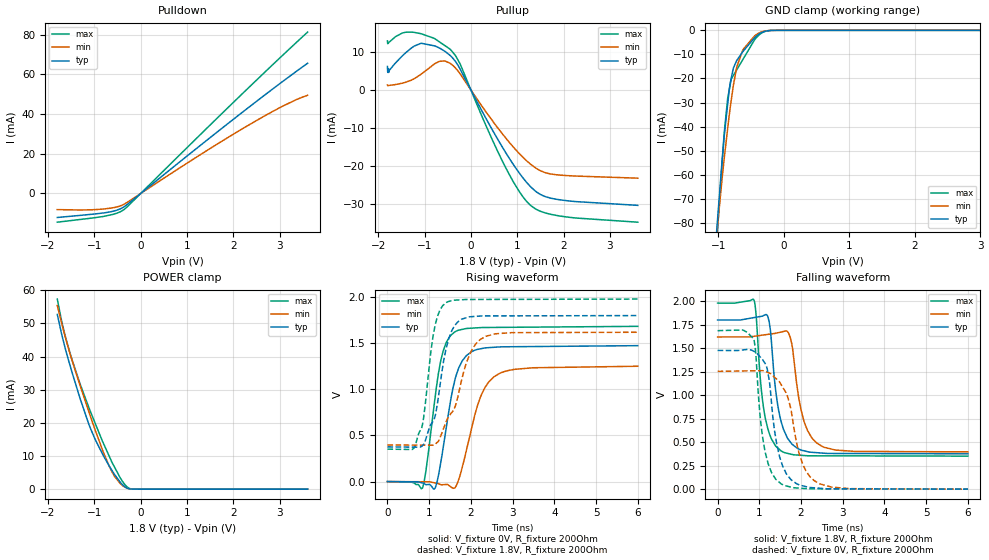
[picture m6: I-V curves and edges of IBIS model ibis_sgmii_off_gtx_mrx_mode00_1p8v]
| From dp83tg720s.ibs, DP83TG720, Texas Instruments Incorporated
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| ibis_sgmii_off_gtx_mrx_mode00_1p8v
[Model]   ibis_sgmii_off_gtx_mrx_mode00_1p8v
Model_type   I/O
Polarity   Non-Inverting
Enable   Active-Low
Vinl = 0.54
Vinh = 1.26
Vmeas = 0.9
Vref = 0.9
Cref = 2pF
Rref = 100000
|   typ   min   max
C_comp   3.96pF   3.91pF   4.01pF
[Voltage Range]   1.8   1.62   1.98
[Temperature Range]   27   150   -40
[Pullup Reference]   1.8   1.62   1.98
[Pulldown Reference]   -0   -0   -0
[Power Clamp Reference]   1.8   1.62   1.98
[GND Clamp Reference]   0   0   0
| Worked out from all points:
|   slope of the pulldown table from 0 to 0.27 V, typ, clamps not added: 52.7 ohm
|   slope of the pullup table from 0 to 0.27 V, typ, clamps not added: 43.2 ohm
|   GND clamp passes 1 mA (typ) near -0.34 V on its own axis
|   POWER clamp passes 1 mA (typ) near -0.37 V on its own axis
|   falling waveform, V_fixture 1.8V, R_fixture 200Ohm: 20-80 % time 263ps typ, 310ps min, 232ps max; typ from 1.8 V to 0.376 V
|   rising waveform, V_fixture 0V, R_fixture 200Ohm: 20-80 % time 357ps typ, 470ps min, 311ps max; typ from 0 V to 1.47 V
|   rising waveform, V_fixture 1.8V, R_fixture 200Ohm: 20-80 % time 343ps typ, 566ps min, 263ps max; typ from 0.376 V to 1.8 V
|   falling waveform, V_fixture 0V, R_fixture 200Ohm: 20-80 % time 293ps typ, 392ps min, 243ps max; typ from 1.48 V to 0 V
[Pulldown]
|   Voltage   I(typ)   I(min)   I(max)
-1.8V     -12.1mA    -8.137mA   -14.48mA
-1.109V   -10.61mA   -8.257mA   -12.56mA
-784.8mV  -9.77mA    -7.8mA     -11.48mA
-514.8mV  -8.428mA   -6.797mA   -9.945mA
-358.2mV  -6.681mA   -5.401mA   -8.065mA
1.165V    21.93mA    17.72mA    26.86mA
2.25V     41.92mA    33.37mA    51.53mA
3.065V    56.45mA    43.99mA    69.67mA
3.6V      65.57mA    49.42mA    81.25mA
[GND Clamp]
|   Voltage   I(typ)   I(min)   I(max)
-1.8V     -413mA     -361.3mA   -461.4mA
-1.022V   -83.06mA   -84.73mA   -87.93mA
-941.4mV  -54.43mA   -61.85mA   -55.74mA
-909mV    -44.33mA   -53.48mA   -43.2mA
-855mV    -30.54mA   -40.73mA   -28.24mA
-801mV    -19.92mA   -29.1mA    -20.25mA
-768.6mV  -15.71mA   -22.89mA   -18.77mA
-714.6mV  -12.42mA   -15.06mA   -16.29mA
-622.8mV  -8.805mA   -8.036mA   -12.09mA
-385.2mV  -1.682mA   -1.218mA   -2.156mA
-185.4mV  -38.16uA   -31.25uA   -36.48uA
3.6V      0A         0A         0A
[Pullup]
|   Voltage   I(typ)   I(min)   I(max)
-1.8V     6.185mA    1.29mA     12.95mA
-1.795V   4.753mA    1.15mA     12.22mA
-1.773V   4.631mA    1.179mA    12.47mA
-1.476V   9.02mA     1.793mA    15.04mA
-1.076V   12.31mA    4.131mA    14.85mA
-682.2mV  11.09mA    7.524mA    12.72mA
-444.6mV  9.078mA    7.03mA     10.73mA
-239.4mV  5.661mA    4.359mA    7.036mA
797.4mV   -17.43mA   -13.36mA   -21.6mA
1.305V    -25.74mA   -19.76mA   -30.62mA
1.845V    -28.85mA   -22.38mA   -33.11mA
3.6V      -30.45mA   -23.28mA   -34.89mA
[POWER Clamp]
|   Voltage   I(typ)   I(min)   I(max)
-1.8V     52.72mA    55.43mA    57.36mA
-1.681V   45.36mA    48.74mA    49.19mA
-1.546V   38.34mA    41.85mA    42.08mA
-1.319V   27.84mA    31.74mA    32.21mA
-1.082V   18.24mA    21.83mA    23.29mA
-979.2mV  14.91mA    17.7mA     19.75mA
-806.4mV  10.12mA    11.14mA    13.88mA
-612mV    5.438mA    5.014mA    7.891mA
-444.6mV  2.133mA    1.733mA    3.461mA
-293.4mV  326.9uA    317uA      674.2uA
-109.8mV  6.028uA    13.64uA    2.638uA
3.6V      0A         0A         0A
[Ramp]
R_load = 200
|   typ   min   max
dV/dt_r   0.883409/3.55174e-10   0.749633/4.67912e-10   1.00891/3.08744e-10
dV/dt_f   0.854249/2.6119e-10   0.733479/3.07972e-10   0.976809/2.29874e-10
[Falling Waveform]
V_fixture = 1.8V
V_fixture_min = 1.62V
V_fixture_max = 1.98V
R_fixture = 200Ohm
C_fixture = 0F
|   Time   V(typ)   V(min)   V(max)
0s        1.8V       1.62V      1.98V
871.6ps   1.825V     1.626V     2.013V
1.129ns   1.852V     1.642V     791.4mV
1.259ns   1.714V     1.65V      569.1mV
1.388ns   1.068V     1.658V     462mV
1.526ns   714.1mV    1.672V     405.8mV
1.74ns    504.1mV    1.617V     374.3mV
1.999ns   417.1mV    846.3mV    360.5mV
2.374ns   388.7mV    492.2mV    355.1mV
6ns       376mV      397.2mV    351.7mV
[Rising Waveform]
V_fixture = 0V
V_fixture_min = 0V
V_fixture_max = 0V
R_fixture = 200Ohm
C_fixture = 0F
|   Time   V(typ)   V(min)   V(max)
0s        51.23uV    46.27uV    80.42uV
837.8ps   -14.76mV   -1.401mV   -70.72mV
926.2ps   -33.48mV   -1.554mV   129.5mV
1.155ns   -56.32mV   -15.29mV   957.1mV
1.338ns   373.6mV    -33.14mV   1.418V
1.609ns   1.086V     -69.26mV   1.62V
1.89ns    1.364V     333.4mV    1.658V
2.226ns   1.438V     911.2mV    1.668V
2.553ns   1.455V     1.135V     1.67V
6ns       1.472V     1.249V     1.682V
[Rising Waveform]
V_fixture = 1.8V
V_fixture_min = 1.62V
V_fixture_max = 1.98V
R_fixture = 200Ohm
C_fixture = 0F
|   Time   V(typ)   V(min)   V(max)
0s        375.9mV    397mV      351.6mV
663.8ps   373.1mV    395.2mV    383mV
856.3ps   397.9mV    394.7mV    659.6mV
1.113ns   664.4mV    398.4mV    1.621V
1.256ns   1.029V     468mV      1.856V
1.405ns   1.437V     646.6mV    1.938V
1.681ns   1.728V     906.5mV    1.967V
1.975ns   1.785V     1.382V     1.973V
2.339ns   1.794V     1.57V      1.973V
6ns       1.798V     1.618V     1.977V
[Falling Waveform]
|Gnd
V_fixture = 0V
V_fixture_min = 0V
V_fixture_max = 0V
R_fixture = 200Ohm
C_fixture = 0F
|   Time   V(typ)   V(min)   V(max)
0s        1.476V     1.253V     1.686V
863.5ps   1.469V     1.26V      1.6V
920.6ps   1.451V     1.26V      1.413V
1.023ns   1.405V     1.261V     763.7mV
1.129ns   1.344V     1.256V     423.8mV
1.526ns   290.3mV    1.11V      55.91mV
1.74ns    111.7mV    884.6mV    24.24mV
2.034ns   36.43mV    273.3mV    8.619mV
2.434ns   10.68mV    59.35mV    3.88mV
6ns       212.7uV    210.1uV    214.5uV
